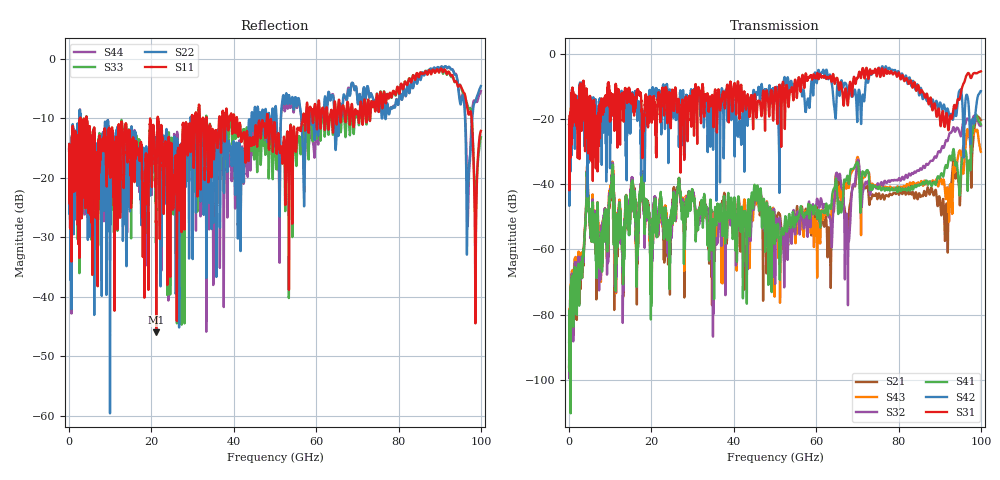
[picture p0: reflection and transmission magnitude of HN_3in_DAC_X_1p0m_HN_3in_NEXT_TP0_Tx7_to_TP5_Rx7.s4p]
# GHz S RI R 45
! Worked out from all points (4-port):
!   4000 points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, 25 MHz to 100 GHz, reference 45 ohm
!   strongest paths, dB at 25 MHz, 25.02 GHz, 50.02 GHz, 75.03 GHz, 100 GHz:
!     S31: -21.6, -11.6, -10.7, -4.8, -5.5
!     S42: -21.7, -14.4, -14.5, -5.1, -11.5
!     S41: -88.4, -48.6, -54.6, -41.5, -21.7
!     S32: -96.1, -49.7, -63.6, -39.8, -22.2
!     S43: -96.2, -50.2, -57.1, -40.6, -30.1
!     S21: -93.7, -48.5, -54.6, -43.8, -20.4
!   lowest |S11| = -45.9 dB at 21.18 GHz (marker M1), VSWR 1.01, Z = 45 - j0.455 ohm
!   |S11| at or under -10 dB: 4.326 GHz to 19.7 GHz (15.37 GHz wide, 128 % of centre); 21.65 GHz to 29.82 GHz (8.168 GHz wide, 31.7 % of centre); 48.29 GHz to 56.77 GHz (8.486 GHz wide, 16.2 % of centre)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
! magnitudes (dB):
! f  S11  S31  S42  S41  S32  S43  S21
! 25 MHz  -15.1  -21.6  -21.7  -88.4  -96.1  -96.2  -93.7
! 4.475 GHz  -12.6  -15.6  -17.7  -38.1  -38.0  -37.7  -38.4
! 21.18 GHz  -45.9  -25.8  -10.8  -52.5  -49.5  -51.2  -50.1
! 67.42 GHz  -8.2  -13.1  -10.1  -38.1  -49.1  -41.0  -55.4
! 70.08 GHz  -8.8  -7.5  -17.0  -33.4  -32.8  -31.7  -34.7
! 91.58 GHz  -2.3  -18.6  -18.2  -34.2  -26.5  -44.1  -46.7
! 100 GHz  -12.1  -5.5  -11.5  -21.7  -22.2  -30.1  -20.4
